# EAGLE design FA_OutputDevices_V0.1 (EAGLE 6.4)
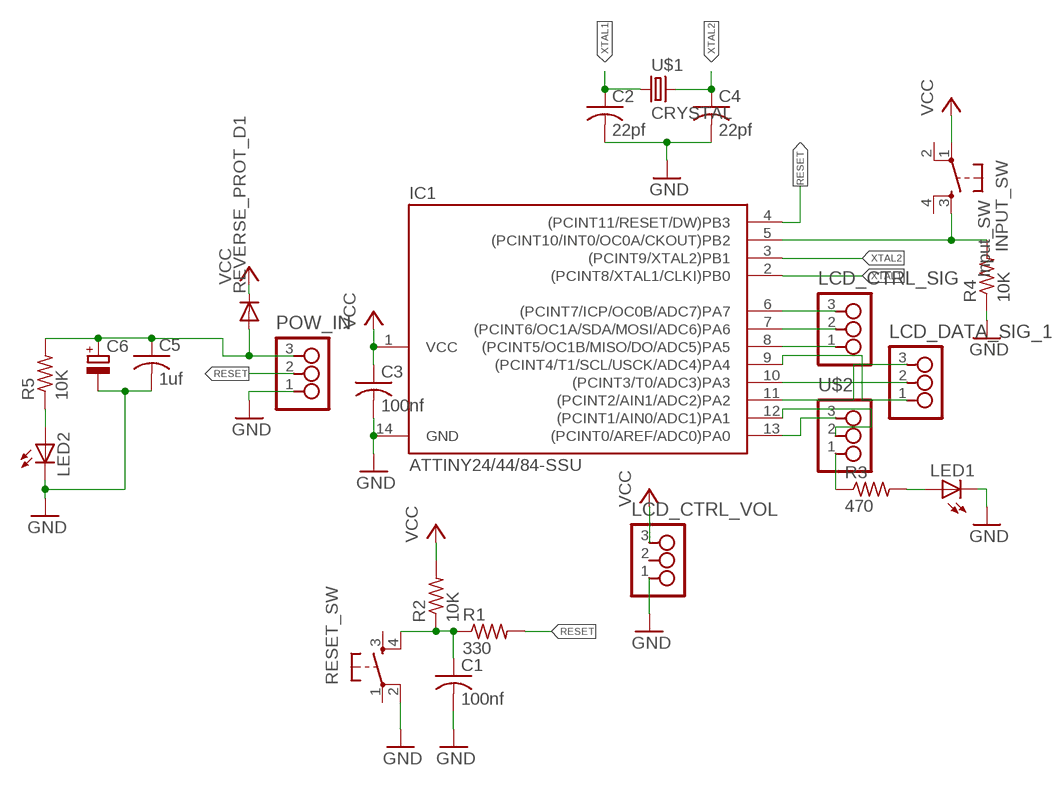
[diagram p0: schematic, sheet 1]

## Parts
C1  100nf  C-USC1206  [C1206]
C2  22pf  C-USC1206  [C1206]
C3  100nf  C-USC1206  [C1206]
C4  22pf  C-USC1206  [C1206]
C5  1uf  C-USC1206  [C1206]
C6  CPOL-EUD  [PANASONIC_D]
IC1  ATTINY24/44/84-SSU  [SOIC14]
INPUT_SW  Input_SW  6MM_SWITCH6MM_SWITCH  [6MM_SWITCH]
LCD_CTRL_SIG  3_PIN_HEADERHEADER  [SMT_PINS_3]
LCD_CTRL_VOL  3_PIN_HEADERHEADER  [SMT_PINS_3]
LCD_DATA_SIG_1  3_PIN_HEADERHEADER  [SMT_PINS_3]
LED1  LEDSMT1206  [1206]
LED2  LEDSMT1206  [1206]
POW_IN  3_PIN_HEADERHEADER  [SMT_PINS_3]
R1  330  R-US_R1206  [R1206]
R2  10K  R-US_R1206  [R1206]
R3  470  R-US_R1206  [R1206]
R4  10K  R-US_R1206  [R1206]
R5  10K  R-US_R1206  [R1206]
RESET_SW  6MM_SWITCH6MM_SWITCH  [6MM_SWITCH]
REVERSE_PROT_D1  DIODESOD123  [SOD123]
U$1  CRYSTAL  [2-SMD-5X3MM]
U$2  3_PIN_HEADERHEADER  [SMT_PINS_3]

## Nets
GND: C1.2 C2.2 C3.2 C4.2 C5.2 C6.- IC1.14(GND) LCD_CTRL_VOL.1 LED1.C LED2.C POW_IN.1 R4.1 RESET_SW.2(P1)
N$1: C1.1 R1.1 R2.1 RESET_SW.4(S1)
N$2: IC1.13((PCINT0/AREF/ADC0)PA0) U$2.3
N$3: IC1.12((PCINT1/AIN0/ADC1)PA1) U$2.2
N$4: LED1.A R3.2
N$5: IC1.8((PCINT5/OC1B/MISO/DO/ADC5)PA5) LCD_CTRL_SIG.1
N$6: IC1.7((PCINT6/OC1A/SDA/MOSI/ADC6)PA6) LCD_CTRL_SIG.2
N$7: IC1.6((PCINT7/ICP/OC0B/ADC7)PA7) LCD_CTRL_SIG.3
N$8: IC1.11((PCINT2/AIN1/ADC2)PA2) LCD_DATA_SIG_1.3
N$9: IC1.10((PCINT3/T0/ADC3)PA3) LCD_DATA_SIG_1.2
N$10: IC1.9((PCINT4/T1/SCL/USCK/ADC4)PA4) LCD_DATA_SIG_1.1
N$11: R3.1 U$2.1
N$12: IC1.5((PCINT10/INT0/OC0A/CKOUT)PB2) INPUT_SW.3(S) R4.2
N$13: C5.1 C6.+ POW_IN.3 R5.2 REVERSE_PROT_D1.ANODE(A)
N$17: LED2.A R5.1
RESET: IC1.4((PCINT11/RESET/DW)PB3) POW_IN.2 R1.2
VCC: C3.1 IC1.1(VCC) INPUT_SW.1(P) LCD_CTRL_VOL.3 R2.2 REVERSE_PROT_D1.CATHODE(C)
XTAL1: C2.1 IC1.2((PCINT8/XTAL1/CLKI)PB0) U$1.P$1
XTAL2: C4.1 IC1.3((PCINT9/XTAL2)PB1) U$1.P$2
Unconnected: INPUT_SW.2(P1) INPUT_SW.4(S1) LCD_CTRL_VOL.2 RESET_SW.1(P) RESET_SW.3(S)

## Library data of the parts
C1-C5 = rcl:C-US: CAPACITOR, American symbol
C6 = rcl:CPOL-EU: POLARIZED CAPACITOR, European symbol
IC1 = 01_attiny24_44_84:ATTINY24/44/84
INPUT_SW RESET_SW = 01_fab:6MM_SWITCH: OMRON SWITCH
LCD_CTRL_SIG LCD_CTRL_VOL LCD_DATA_SIG_1 POW_IN U$2 = 01_FAB_Hello:3_PIN_HEADER: 3 SMT pin pads
LED1 LED2 = led:LED: LED
R1-R5 = rcl:R-US_: RESISTOR, American symbol
REVERSE_PROT_D1 = 01_fab:DIODE: DIODE
U$1 = fab:CRYSTAL

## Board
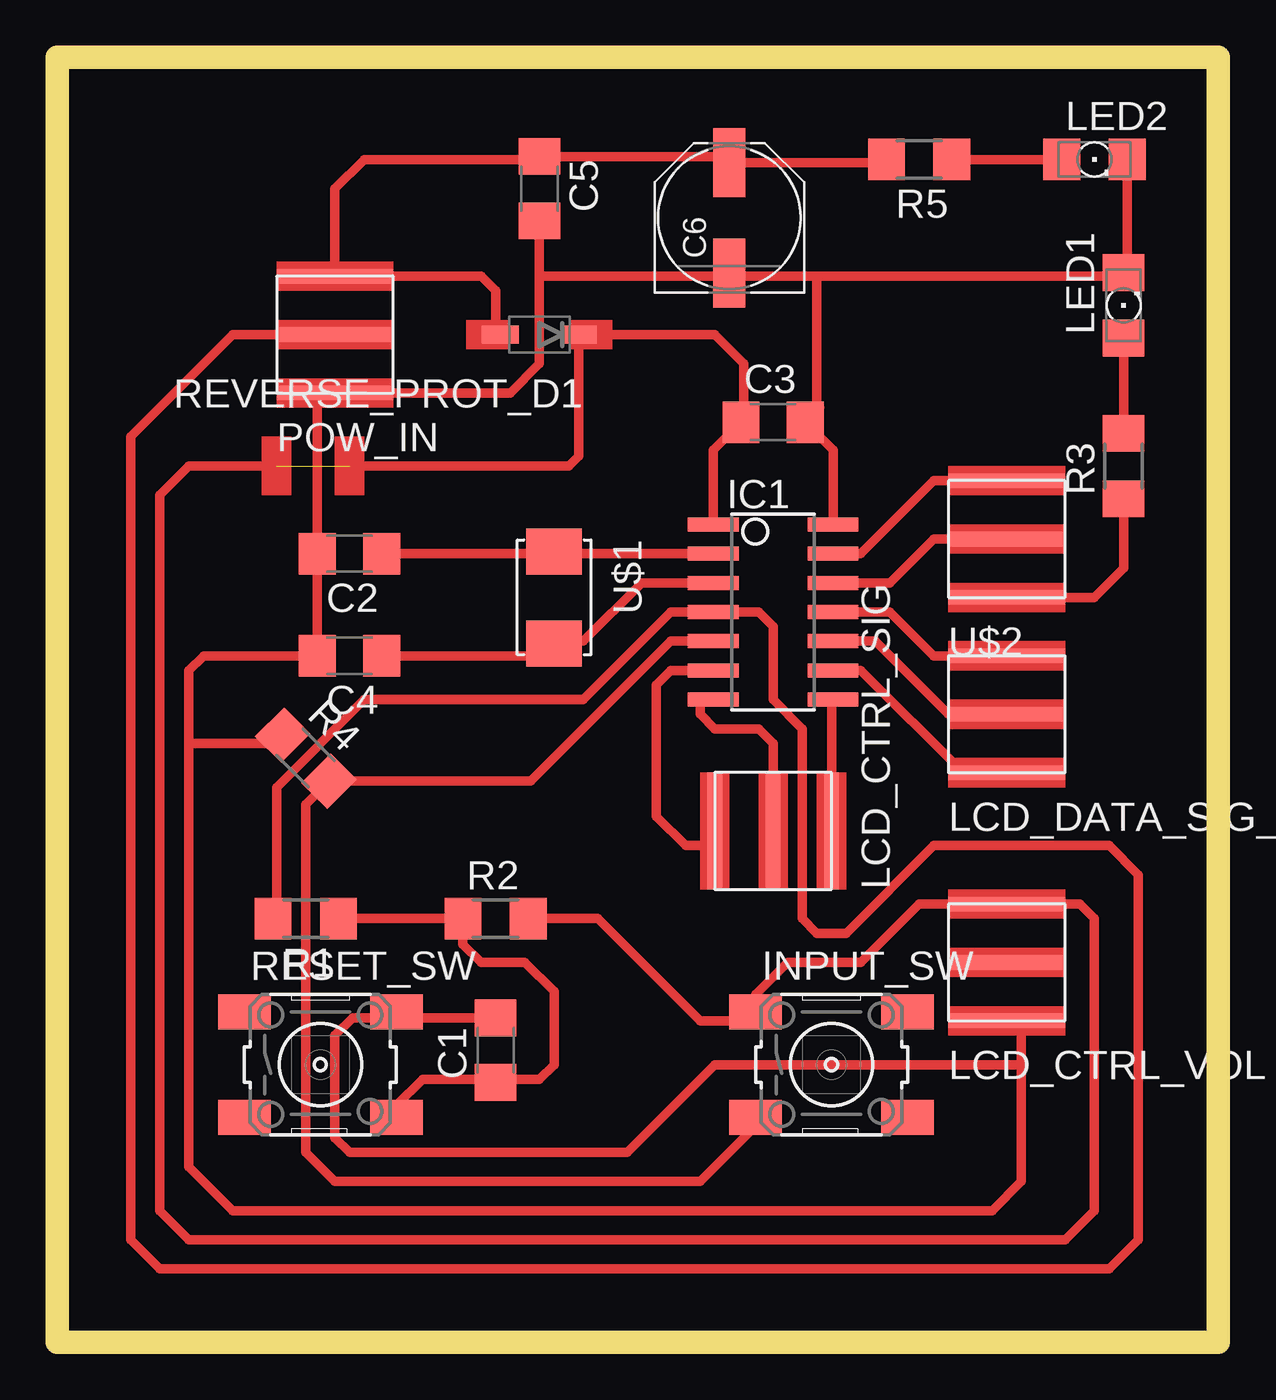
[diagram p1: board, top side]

Size 50.47 x 55.87 mm. Coordinates in mm from the lower left corner, seen from the top.
Outline: 0,0 50.47,0 50.47,55.87 0,55.87 0,0
Copper layers (1*16): Top 0.035mm / dielectric 1.5mm / Bottom 0.035mm
Design rules "default *": minimum track width 16mil, minimum drill 24mil, track to track 12mil, track to pad 12mil, pad to pad 8mil, via to via 8mil, smd to smd 8mil, copper to edge 40mil, drill to drill 8mil, minimum pad ring 10mil, minimum via ring 8mil, stop-mask expansion 4mil, vias tented up to drill 0mil, thermal gap 10mil

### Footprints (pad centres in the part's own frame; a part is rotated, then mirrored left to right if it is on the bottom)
C1206 = smd 1.6 x 1.8: 1 -1.4,0; 2 1.4,0
PANASONIC_D = smd 3 x 1.4: + 2.4,0; - -2.4,0
SOIC14 = smd 0.61 x 2.21: 1 -3.81,-2.603; 2 -2.54,-2.603; 3 -1.27,-2.603; 4 0,-2.603; 5 1.27,-2.603; 6 2.54,-2.603; 7 3.81,-2.603; 8 3.81,2.603; 9 2.54,2.603; 10 1.27,2.603; 11 0,2.603; 12 -1.27,2.603; 13 -2.54,2.603; 14 -3.81,2.603
6MM_SWITCH = smd 2.286 x 1.524: 1 -3.302,2.286; 2 3.302,2.286; 3 -3.302,-2.286; 4 3.302,-2.286
SMT_PINS_3 = smd 5.08 x 0.635: 1 0,0; 2 0,2.54; 3 0,5.08
1206 = smd 1.6 x 1.803: A -1.422,0; C 1.422,0
R1206 = smd 1.6 x 1.803: 1 -1.422,0; 2 1.422,0
SOD123 = smd 1.6 x 0.8: ANODE 1.7,0; CATHODE -1.7,0
2-SMD-5X3MM = smd 2 x 2.4: P$1 -2,0; P$2 2,0

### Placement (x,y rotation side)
C1  19.05,12.7 90 top
C2  12.7,34.29 180 top
C3  31.11,40.01 0 top
C4  12.7,29.84 180 top
C5  20.95,50.16 270 top
C6  29.21,48.9 90 top
IC1  31.11,31.75 270 top
INPUT_SW  33.66,12.06 0 top
LCD_CTRL_SIG  33.66,22.23 90 top
LCD_CTRL_VOL  41.27,13.97 0 top
LCD_DATA_SIG_1  41.27,24.77 0 top
LED1  46.35,45.09 90 top
LED2  45.09,51.44 0 top
POW_IN  12.06,41.27 0 top
R1  10.79,18.41 180 top
R2  19.05,18.41 0 top
R3  46.35,38.1 90 top
R4  10.79,25.4 315 top
R5  37.47,51.44 180 top
RESET_SW  11.43,12.06 0 top
REVERSE_PROT_D1  20.95,43.81 180 top
U$1  21.59,32.38 270 top
U$2  41.27,32.38 0 top

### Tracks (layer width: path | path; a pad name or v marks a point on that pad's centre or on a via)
GND
  Top 0.406: C2.2 C4.2 6.35,29.84 5.71,29.21 5.71,26.04 | C2.2 11.3,34.8 11.43,34.92 11.43,34.42 C2.2 | IC1.14 33.72,38.8 C3.2 33.15,40.64 33.02,40.64 33.02,46.35 | 20.95,46.35 20.95,42.55 19.68,41.27 POW_IN.1 11.43,41.27 11.3,41.15 C2.2 | 20.95,46.35 C5.2 | C1.2 14.98,14.1 | 14.98,14.1 RESET_SW.2 | 9.26,26.41 R4.1 9.42,26.04 5.71,26.04 | 5.71,26.04 5.71,7.62 7.62,5.71 40.64,5.71 41.91,6.99 41.91,12.06 | 14.98,14.1 12.83,14.1 12.06,13.34 12.06,8.89 12.7,8.26 24.77,8.26 28.57,12.06 41.91,12.06 | 41.91,12.06 41.91,13.97 LCD_CTRL_VOL.1 | 33.02,46.35 29.35,46.35 C6.- 29.07,46.35 20.95,46.35 | 33.02,46.35 46.35,46.35 LED1.C 46.51,46.51 LED2.C
N$1
  Top 0.406: R1.1 R2.1 17.63,17.3 18.41,16.51 20.32,16.51 21.59,15.24 21.59,12.06 20.95,11.43 19.18,11.43 C1.1 18.92,11.43 15.88,11.43 14.73,10.29 RESET_SW.4
N$2
  Top 0.406: IC1.13 34.92,34.29 38.1,37.47 U$2.3
N$3
  Top 0.406: IC1.12 36.2,33.02 38.1,34.92 U$2.2
N$4
  Top 0.406: LED1.A R3.2
N$5
  Top 0.406: IC1.8 33.66,27.88 LCD_CTRL_SIG.1
N$6
  Top 0.406: LCD_CTRL_SIG.2 31.11,26.04 30.48,26.67 28.57,26.67 27.94,27.3 27.94,27.94 IC1.7
N$7
  Top 0.406: IC1.6 26.67,29.21 26.04,28.57 26.04,22.86 27.3,21.59 28.57,21.59 LCD_CTRL_SIG.3
N$8
  Top 0.406: IC1.11 36.2,31.75 38.1,29.84 LCD_DATA_SIG_1.3
N$9
  Top 0.406: 39.37,27.3 LCD_DATA_SIG_1.2 38.73,27.3 35.56,30.48 IC1.10
N$10
  Top 0.406: IC1.9 34.92,29.21 39.37,24.77 LCD_DATA_SIG_1.1
N$11
  Top 0.406: R3.1 46.35,33.66 45.09,32.38 U$2.1
N$12
  Top 0.406: IC1.5 26.67,30.48 20.58,24.39 R4.2 10.79,23.39 10.79,8.26 12.06,6.99 27.94,6.99 30.35,9.4 INPUT_SW.3
N$13
  Top 0.406: R5.2 35.9,51.3 C6.+ 28.94,51.56 C5.1 20.82,51.44 13.34,51.44 12.06,50.16 POW_IN.3 18.41,46.35 19.05,45.72 19.05,44.02 REVERSE_PROT_D1.ANODE
N$17
  Top 0.406: R5.1 LED2.A
RESET
  Top 0.406: R1.2 9.53,18.57 9.53,24.13 13.34,27.94 22.86,27.94 26.67,31.75 IC1.4 30.48,31.75 31.11,31.11 31.11,27.94 32.38,26.67 32.38,18.41 33.02,17.78 34.29,17.78 38.1,21.59 45.72,21.59 46.99,20.32 46.99,4.45 45.72,3.17 4.45,3.17 3.17,4.45 3.17,39.37 7.62,43.81 POW_IN.2
VCC  (1 unrouted)
  Top 0.406: IC1.1 28.51,38.8 C3.1 29.84,40.13 29.84,42.55 28.57,43.81 REVERSE_PROT_D1.CATHODE 22.66,38.53 22.23,38.1 12.7,38.1 | R2.2 23.5,18.41 27.94,13.97 29.97,13.97 INPUT_SW.1 30.35,15.11 31.75,16.51 34.92,16.51 37.47,19.05 LCD_CTRL_VOL.3 44.45,19.05 45.09,18.41 45.09,5.71 43.81,4.45 5.71,4.45 4.45,5.71 4.45,36.83 5.71,38.1 9.53,38.1
XTAL1
  Top 0.406: IC1.2 21.59,34.29 U$1.P$1 21.5,34.29 C2.1
XTAL2
  Top 0.406: IC1.3 25.4,33.02 22.86,30.48 21.68,30.48 U$1.P$2 21.05,29.84 C4.1
(copper drawn outside any net)
  shapes: Top area x19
